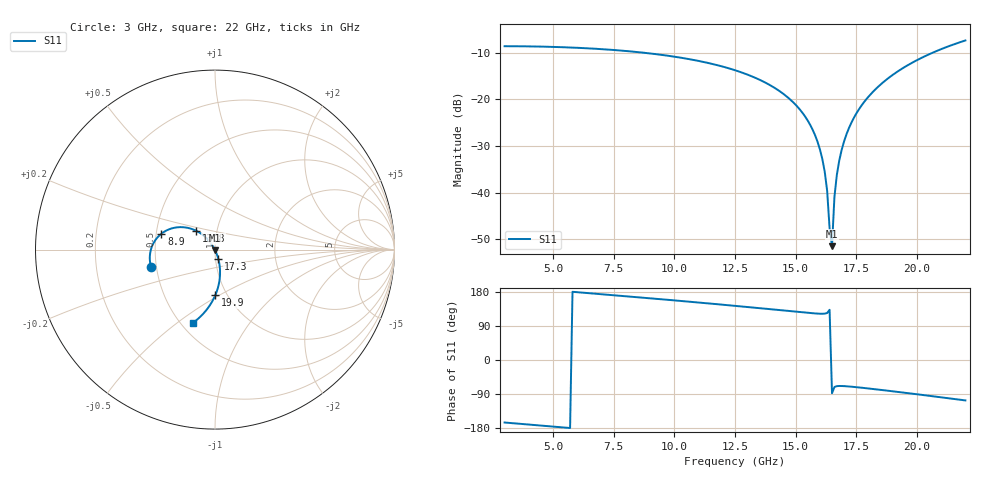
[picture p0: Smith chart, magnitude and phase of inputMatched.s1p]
! AWR Design Environment (7628) Thu Jan 14 16:43:17 2016
! Document = 'inputMatched'
! nPorts: 1, nXvals: 191
# HZ S MA R 50
!Freq MagS11 AngS11
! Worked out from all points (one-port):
!   191 points, 3 GHz to 22 GHz, reference 50 ohm
!   lowest |S11| = -51.5 dB at 16.5 GHz (marker M1), VSWR 1.01, Z = 50 - j0.266 ohm
!   |S11| at or under -10 dB: 8.651 GHz to 20.67 GHz (12.02 GHz wide, 82 % of centre)
!   S11 on the Smith chart (normalised r, x): 3 GHz: 0.47, -0.10; 8.9 GHz: 0.53, +0.11; 13.8 GHz: 0.79, +0.17; 17.3 GHz: 1.03, -0.11; 19.9 GHz: 0.88, -0.48; 22 GHz: 0.57, -0.57
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3e9  0.3694 -165.0
5.4e9  0.3604 -177.9
7.8e9  0.3317 169.3
8.9e9  0.3111 163.4
1.02e10  0.28 156.2
1.25e10  0.2043 142.9
1.38e10  0.1482 135.0
1.49e10  0.09256 128.1
1.53e10  0.07038 125.7
1.56e10  0.05306 123.9
1.58e10  0.04119 122.9
1.6e10  0.02906 122.1
1.62e10  0.01668 122.4
1.63e10  0.01041 123.9
1.64e10  0.004144 132.5
1.65e10  0.002661 -87.9
1.66e10  0.008975 -71.3
1.67e10  0.01549 -69.0
1.68e10  0.02209 -68.5
1.69e10  0.02875 -68.6
1.71e10  0.04227 -69.3
1.73e10  0.05604 -70.4
1.77e10  0.08427 -73.0
1.82e10  0.1208 -76.5
1.89e10  0.174 -81.8
1.97e10  0.2373 -88.0
1.99e10  0.2535 -89.6
2.2e10  0.4257 -106.7
